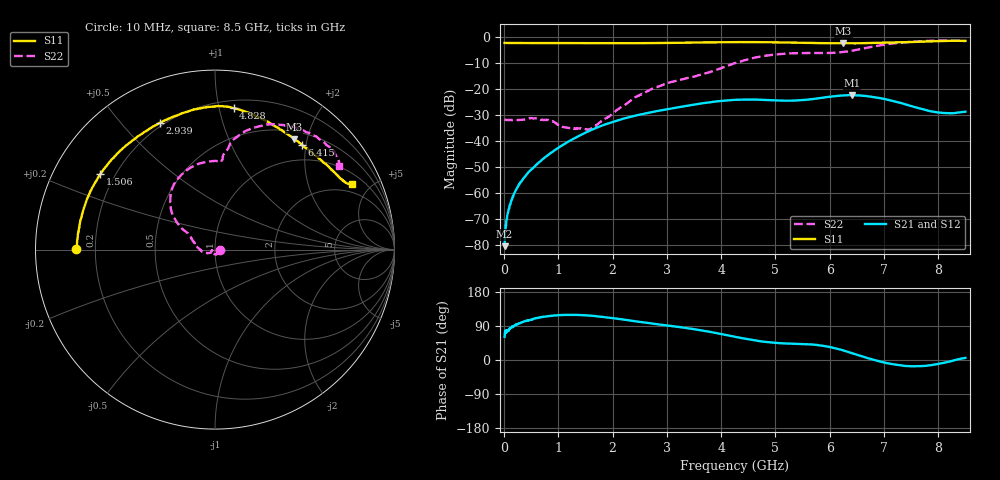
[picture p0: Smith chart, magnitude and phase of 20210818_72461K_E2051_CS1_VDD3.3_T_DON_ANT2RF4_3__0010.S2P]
!Agilent Technologies,E5071C,MY46417908,A.11.23
!Date: Wed Aug 18 14:33:13 2021
!Data & Calibration Information:
!Freq	S11:SOLT2(ON)	S21:SOLT2(ON)	S12:SOLT2(ON)	S22:SOLT2(ON)
!PortZ  Port1:50+j0  Port2:50+j0
!Above PortZ is port z conversion or system Z0 setting when saving the data.
!When reading, reference impedance value at option line is always used.
# Hz S dB R 50
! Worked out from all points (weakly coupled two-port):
!   1601 points, 10 MHz to 8.5 GHz, reference 50 ohm
!   highest |S21| = -22.37 dB at 6.409 GHz (marker M1); lowest = -80.6 dB at 10 MHz (marker M2)
!   lowest |S11| = -2.4 dB at 6.25 GHz (marker M3), VSWR 7.19, Z = 31 + j88.9 ohm
!   |S11| at or under -10 dB: nowhere
!   |S22| runs from -35.6 to -1.3 dB; largest |S21 - S12| = 0.00033
!   S11 on the Smith chart (normalised r, x): 10 MHz: 0.13, +0.00; 1.506 GHz: 0.15, +0.29; 2.939 GHz: 0.18, +0.64; 4.828 GHz: 0.26, +1.11; 6.415 GHz: 0.69, +1.92; 8.5 GHz: 1.50, +3.88
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1e7  -2.23 179.7  -80.57 61.3  -81.84 93.7  -31.65 -2.5
6.836875e7  -2.27 178.4  -67.77 77.3  -67.80 76.7  -31.94 -9.0
1.214312e8  -2.27 177.1  -63.80 84.9  -63.89 84.4  -31.93 -15.5
2.169438e8  -2.29 174.9  -59.05 93.1  -58.87 92.9  -31.96 -28.4
3.336812e8  -2.29 172.3  -55.08 99.8  -55.16 99.3  -31.90 -47.5
7.52875e8  -2.31 162.9  -46.36 114.7  -46.38 114.6  -31.94 -101.6
1.097781e9  -2.32 155.5  -41.39 118.8  -41.38 119.0  -34.66 -143.0
1.426769e9  -2.33 148.5  -37.59 118.4  -37.60 118.4  -35.22 -168.7
1.506362e9  -2.34 146.7  -36.79 118.0  -36.80 117.9  -35.48 -166.1
1.649631e9  -2.34 143.7  -35.42 116.3  -35.42 116.3  -34.79 -160.3
2.424344e9  -2.36 125.7  -30.25 102.1  -30.25 102.1  -23.15 -171.1
2.843538e9  -2.29 115.8  -28.42 93.9  -28.42 93.9  -19.02 165.9
2.93905e9  -2.28 113.7  -28.07 92.3  -28.07 92.3  -18.33 161.4
4.255e9  -1.96 90.0  -24.18 61.4  -24.19 61.4  -10.06 139.8
4.828075e9  -1.99 82.5  -24.26 47.7  -24.27 47.7  -7.14 119.6
5.671769e9  -2.26 67.8  -23.93 40.9  -23.93 41.0  -6.12 89.9
6.25015e9  -2.43 54.4  -22.51 25.3  -22.52 25.3  -5.74 85.2
6.409338e9  -2.38 50.6  -22.37 18.2  -22.39 18.2  -5.27 84.0
6.414644e9  -2.39 50.4  -22.37 17.9  -22.39 17.9  -5.25 83.9
7.088538e9  -2.10 35.9  -24.23 -9.3  -24.27 -9.5  -2.68 69.7
7.926925e9  -1.61 26.2  -28.83 -12.2  -28.81 -12.2  -1.39 45.0
8.5e9  -1.44 25.5  -28.75 5.6  -28.77 5.4  -1.58 34.1
